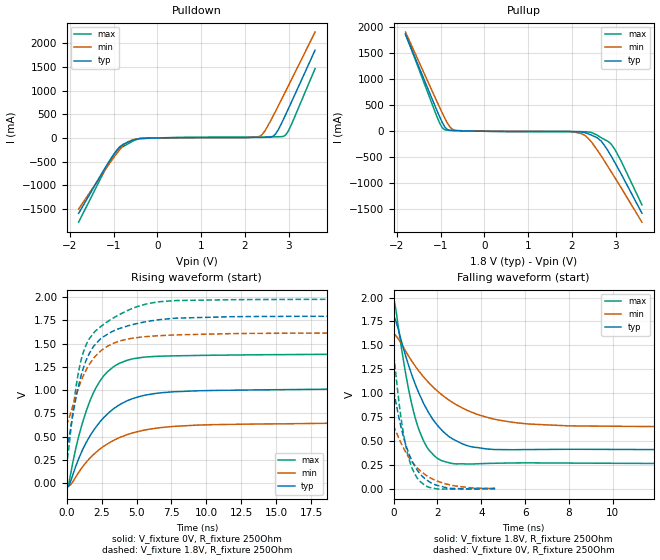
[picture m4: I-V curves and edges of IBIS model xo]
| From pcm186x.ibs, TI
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|   xo Model
[Model]   xo
Model_type   Output
Polarity   Inverting
Vmeas = 0.9
Vref = 0
Cref = 2pF
Rref = 400
|   typ   min   max
|   (nom PVT)   (fast PVT)   (slow PVT)
C_comp   9.427e-12   9.427e-12   9.543e-12
| Where nom  PVT is Nominal Process, 1.8V, 27C
|   Fast PVT is Strong Process,  1.98V, -40C
|   Slow PVT is Weak Process,   1.62V, 125C
[Voltage Range]   1.8   1.62   1.98
|Junction Temperature
[Temperature Range]   27   125   -40
[Pullup Reference]   1.8   1.62   1.98
[Pulldown Reference]   0   0   0
[Power Clamp Reference]   1.8   1.62   1.98
[GND Clamp Reference]   0   0   0
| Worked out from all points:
|   slope of the pulldown table from 0 to 0.27 V, typ, clamps not added: 66.6 ohm
|   slope of the pullup table from 0 to 0.27 V, typ, clamps not added: 143 ohm
|   falling waveform, V_fixture 1.8V, R_fixture 250Ohm: 20-80 % time 1.54ns typ, 2.6ns min, 927ps max; typ from 1.8 V to 0.406 V
|   rising waveform, V_fixture 0V, R_fixture 250Ohm: 20-80 % time 2.75ns typ, 3.33ns min, 1.92ns max; typ from 0.001 V to 1.01 V
|   rising waveform, V_fixture 1.8V, R_fixture 250Ohm: 20-80 % time 1.84ns typ, 2.01ns min, 1.74ns max; typ from 0.405 V to 1.8 V
|   falling waveform, V_fixture 0V, R_fixture 250Ohm: 20-80 % time 875ps typ, 1.3ns min, 599ps max; typ from 1.01 V to 0.002 V
[Pulldown]
|   Voltage   I(typ)   I(min)   I(max)
-1.8V     -1.594A    -1.503A    -1.779A
-1.001V   -352.1mA   -416.9mA   -362.7mA
-851.6mV  -179.7mA   -237.5mA   -211.8mA
-559.1mV  -48.21mA   -37.8mA    -64.73mA
75.6mV    1.269mA    674.1uA    2.193mA
1.981V    9.385mA    5.095mA    16.74mA
2.38V     12.4mA     60.86mA    17.23mA
2.578V    18.75mA    348.6mA    20.79mA
2.696V    80.9mA     561.7mA    24.19mA
2.927V    490.5mA    984.7mA    61.56mA
3.067V    770.4mA    1.243A     296.4mA
3.6V      1.854A     2.236A     1.464A
[Pullup]
|   Voltage   I(typ)   I(min)   I(max)
-1.8V     1.86A      1.905A     1.872A
-1.071V   378mA      552mA      259.1mA
-916.9mV  104.3mA    276.8mA    34.84mA
-779.4mV  15.75mA    78.29mA    18.49mA
-654.7mV  10.01mA    12.85mA    13.87mA
1.924V    -4.756mA   -3.607mA   -8.089mA
2.263V    -18.23mA   -62.86mA   -8.272mA
2.445V    -73.41mA   -204.3mA   -23.62mA
2.675V    -192.5mA   -480.8mA   -126.2mA
2.888V    -463.5mA   -764.2mA   -237.5mA
3.124V    -817.3mA   -1.084A    -571.1mA
3.6V      -1.575A    -1.747A    -1.414A
[Ramp]
R_load = 250
|   typ   min   max
dV/dt_r   0.60717/2.7454e-09   0.387146/3.32709e-09   0.831043/1.92038e-09
dV/dt_f   0.836364/1.54892e-09   0.586358/2.62949e-09   1.02922/9.26232e-10
[Falling Waveform]
V_fixture = 1.8V
V_fixture_min = 1.62V
V_fixture_max = 1.98V
R_fixture = 250Ohm
|   Time   V(typ)   V(min)   V(max)
0s        1.8V       1.62V      1.98V
100ps     1.752V     1.603V     1.877V
575ps     1.37V      1.429V     1.171V
1.035ns   1.066V     1.268V     703.4mV
1.5ns     836.5mV    1.136V     444.5mV
2.16ns    623.9mV    991.8mV    298.8mV
2.71ns    520.4mV    900.8mV    265.1mV
3.55ns    441mV      802.5mV    260.7mV
6.27ns    412.4mV    677.7mV    272.8mV
22.15ns   406.4mV    645.8mV    263.3mV
[Rising Waveform]
V_fixture = 0V
V_fixture_min = 0V
V_fixture_max = 0V
R_fixture = 250Ohm
|   Time   V(typ)   V(min)   V(max)
0s        785.5uV    773.9uV    714uV
5ps       -55.64mV   -49.19mV   -64.12mV
120ps     -31.77mV   -32.38mV   -18.74mV
875ps     271.1mV    120.8mV    514.9mV
1.855ns   553.3mV    299.5mV    953.5mV
2.665ns   707.5mV    398.5mV    1.157V
3.75ns    840.2mV    488.3mV    1.287V
5.305ns   935.3mV    562.2mV    1.35V
7.465ns   980.5mV    608.1mV    1.368V
19.95ns   1.013V     646mV      1.386V
[Rising Waveform]
V_fixture = 1.8V
V_fixture_min = 1.62V
V_fixture_max = 1.98V
R_fixture = 250Ohm
|   Time   V(typ)   V(min)   V(max)
0s        404.6mV    641.4mV    263.1mV
5ps       378.4mV    630.6mV    219.6mV
90ps      439.3mV    669.7mV    310.6mV
790ps     1.01V      1.003V     1.153V
1.115ns   1.202V     1.131V     1.374V
1.47ns    1.348V     1.24V      1.515V
2.46ns    1.558V     1.425V     1.686V
4.845ns   1.709V     1.561V     1.887V
7.89ns    1.774V     1.594V     1.963V
29.85ns   1.799V     1.619V     1.978V
[Falling Waveform]
V_fixture = 0V
V_fixture_min = 0V
V_fixture_max = 0V
R_fixture = 250Ohm
|   Time   V(typ)   V(min)   V(max)
0s        1.013V     645.8mV    1.386V
35ps      985.8mV    638.6mV    1.343V
280ps     704mV      508.2mV    839.8mV
490ps     511.8mV    409.6mV    523.5mV
605ps     427mV      363.4mV    396.9mV
770ps     327.4mV    305.6mV    262.3mV
1.095ns   191.7mV    216.5mV    107.8mV
1.54ns    89.43mV    134.5mV    23.75mV
2.34ns    16.7mV     56.5mV     -126.9uV
4.63ns    2.004mV    3.231mV    7.249mV
